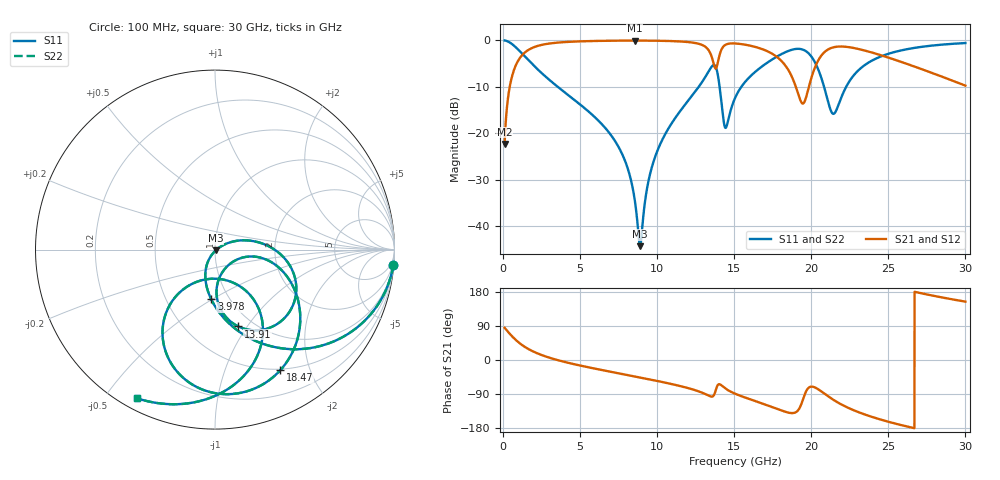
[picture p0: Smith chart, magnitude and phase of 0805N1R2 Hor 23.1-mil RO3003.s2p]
# GHz S MA R 50
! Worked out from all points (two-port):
!   3201 points, 100 MHz to 30 GHz, reference 50 ohm
!   highest |S21| = -0.05 dB at 8.556 GHz (marker M1); lowest = -22.3 dB at 100 MHz (marker M2)
!   |S21| within 3 dB of the highest: 1.273 GHz to 13.48 GHz (12.21 GHz wide, 165 % of centre); 20.71 GHz to 24.38 GHz (3.671 GHz wide, 16.3 % of centre)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
!   lowest |S11| = -44.2 dB at 8.892 GHz (marker M3), VSWR 1.01, Z = 50.4 - j0.447 ohm
!   |S11| at or under -10 dB: 3.553 GHz to 12.69 GHz (9.141 GHz wide, 113 % of centre); 14.05 GHz to 15.46 GHz (1.407 GHz wide, 9.54 % of centre); 20.83 GHz to 22.26 GHz (1.43 GHz wide, 6.64 % of centre)
!   |S22| runs from -44.2 to 0.0 dB; largest |S21 - S12| = 0
!   S11 on the Smith chart (normalised r, x): 100 MHz: 1, -23; 3.978 GHz: 0.82, -0.50; 13.91 GHz: 0.85, -0.91; 18.47 GHz: 0.48, -1.57; 30 GHz: 0.05, -0.60
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0.1  0.997 -4.9  0.07697 85.0  0.07697 85.0  0.997 -4.9
0.47375  0.9389 -22.6  0.3438 67.3  0.3438 67.3  0.9389 -22.6
1.053063  0.7735 -44.9  0.6327 45.1  0.6327 45.1  0.7735 -44.9
2.230375  0.4901 -72.3  0.8695 17.5  0.8695 17.5  0.4901 -72.3
3.977656  0.2781 -94.3  0.9573 -4.9  0.9573 -4.9  0.2781 -94.3
5.089563  0.1989 -104.3  0.9762 -15.4  0.9762 -15.4  0.1989 -104.3
7.490906  0.07171 -121.0  0.9921 -35.0  0.9921 -35.0  0.07171 -121.0
8.556094  0.01871 -115.3  0.9937 -43.5  0.9937 -43.5  0.01871 -115.3
8.892469  0.006146 -46.1  0.9935 -46.1  0.9935 -46.1  0.006146 -46.1
10.06978  0.06857 27.8  0.9897 -55.8  0.9897 -55.8  0.06857 27.8
12.46178  0.2806 5.7  0.9367 -79.6  0.9367 -79.6  0.2806 5.7
13.42419  0.4895 -22.8  0.74 -95.8  0.74 -95.8  0.4895 -22.8
13.91006  0.4471 -73.2  0.5537 -67.6  0.5537 -67.6  0.4471 -73.2
14.42397  0.1146 -51.0  0.8938 -75.1  0.8938 -75.1  0.1146 -51.0
15.05  0.2395 -9.9  0.9258 -88.9  0.9258 -88.9  0.2395 -9.9
18.46981  0.7644 -61.6  0.4926 -138.5  0.4926 -138.5  0.7644 -61.6
19.43222  0.797 -91.0  0.2094 -107.6  0.2094 -107.6  0.797 -91.0
20.03956  0.6577 -113.3  0.412 -70.3  0.412 -70.3  0.6577 -113.3
21.44112  0.1622 -90.1  0.8419 -105.3  0.8419 -105.3  0.1622 -90.1
22.94547  0.4566 -55.5  0.8152 -135.8  0.8152 -135.8  0.4566 -55.5
25.01978  0.7182 -76.8  0.6511 -163.2  0.6511 -163.2  0.7182 -76.8
30  0.9351 -117.6  0.3262 154.0  0.3262 154.0  0.9351 -117.6
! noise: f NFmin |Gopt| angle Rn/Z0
0.1  0.00129  0.9556  1.378  0.006548
3.417  0.007584  0.7476  19  0.005885
6.743  0.01321  0.7225  35.7  0.008576
10.06  0.02062  0.7385  51.69  0.01285
13.39  0.1081  0.9283  67.56  0.2313
16.7  0.06755  0.865  82.26  0.06118
20.03  0.3456  0.9672  96.99  1.05
23.35  0.09957  0.8756  110.3  0.05695
26.67  0.09439  0.855  122.7  0.03261
30  0.1114  0.8655  134.8  0.02704
